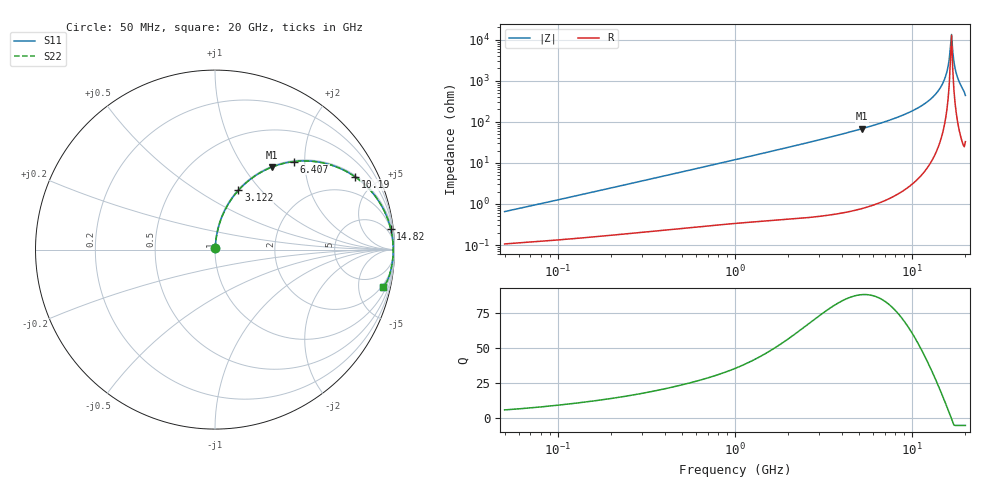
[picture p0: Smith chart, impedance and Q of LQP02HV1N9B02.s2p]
!Murata Part Number: LQP02HV1N9B02
!These Parameters are Measured in Series Mode Connection
!  o--[Z]--o
!Port1  Port2
!  o-------o
!Freq. Start=50[MHz] Stop=20[GHz], 401[Steps]
# Hz S RI R 50
!Freq.(Hz) S11(Real) S11(Imag) S21(Real) S21(Imag) S12(Real) S12(Imag) S22(Real) S22(Imag)
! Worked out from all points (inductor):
!   401 points, 50 MHz to 20 GHz, reference 50 ohm
!   read as one part in series: L = 2.03 nH near 51.52 MHz
!   highest Q = 88 at 5.195 GHz (marker M1), where L = 2.07 nH
!   self-resonance near 16.46 GHz
!   S11 on the Smith chart (normalised r, x): 50 MHz: 1.00, +0.01; 3.122 GHz: 1.01, +0.76; 6.407 GHz: 1.02, +1.77; 10.19 GHz: 1.06, +3.82; 14.82 GHz: 2, +16; 20 GHz: 1.66, -8.75
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5e7  0.00111 0.00643  0.9989 -0.00643  0.9989 -0.00643  0.00111 0.00643
1.364002e8  0.00177 0.0169  0.9982 -0.0169  0.9982 -0.0169  0.00177 0.0169
3.721004e8  0.00423 0.0447  0.9958 -0.0447  0.9958 -0.0447  0.00423 0.0447
1e9  0.0172 0.1168  0.9828 -0.1168  0.9828 -0.1168  0.0172 0.1168
2.728004e9  0.1019 0.2954  0.8981 -0.2954  0.8981 -0.2954  0.1019 0.2954
3.121702e9  0.1302 0.3299  0.8698 -0.3299  0.8698 -0.3299  0.1302 0.3299
5.194772e9  0.3164 0.4594  0.6836 -0.4594  0.6836 -0.4594  0.3164 0.4594
6.406762e9  0.4397 0.4906  0.5603 -0.4906  0.5603 -0.4906  0.4397 0.4906
7.442007e9  0.5439 0.4919  0.4561 -0.4919  0.4561 -0.4919  0.5439 0.4919
1.019291e10  0.7814 0.4049  0.2186 -0.4049  0.2186 -0.4049  0.7814 0.4049
1.276073e10  0.9227 0.2533  0.0773 -0.2533  0.0773 -0.2533  0.9227 0.2533
1.396067e10  0.9609 0.1743  0.0391 -0.1743  0.0391 -0.1743  0.9609 0.1743
1.482269e10  0.9786 0.1174  0.0214 -0.1174  0.0214 -0.1174  0.9786 0.1174
1.550395e10  0.9873 0.0732  0.0127 -0.0732  0.0127 -0.0732  0.9873 0.0732
1.573793e10  0.9894 0.0583  0.0106 -0.0583  0.0106 -0.0583  0.9894 0.0583
1.621653e10  0.9921 0.0282  0.00795 -0.0282  0.00795 -0.0282  0.9921 0.0282
1.670968e10  0.9929 -0.00218  0.00709 0.00218  0.00709 0.00218  0.9929 -0.00218
1.696185e10  0.9926 -0.0174  0.00737 0.0174  0.00737 0.0174  0.9926 -0.0174
1.721783e10  0.9919 -0.0326  0.00812 0.0326  0.00812 0.0326  0.9919 -0.0326
1.747767e10  0.9907 -0.0479  0.00934 0.0479  0.00934 0.0479  0.9907 -0.0479
1.800918e10  0.9868 -0.0784  0.0132 0.0784  0.0132 0.0784  0.9868 -0.0784
2e10  0.9365 -0.2092  0.0635 0.2092  0.0635 0.2092  0.9365 -0.2092
